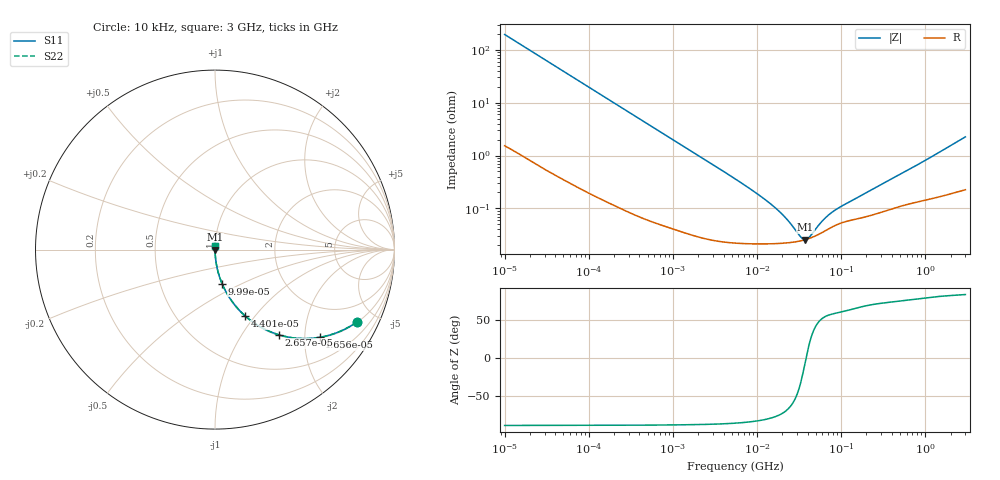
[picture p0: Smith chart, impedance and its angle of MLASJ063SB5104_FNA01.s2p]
! MLASJ063SB5104_FNA01  S-PARAMETER MODEL  ( Standard Model )
! Model Generated by TAIYO YUDEN Corporation (http://www.ty-top.com)
! Version 1.0
! TAIYO YUDEN Control No. 220601
! Copyright(c) 2005 TAIYO YUDEN CO.,LTD. All Rights Reserved.
! Product Description (link to TY-COMPAS)
! https://ds.yuden.co.jp/TYCOMPAS/or/detail?pn=MLASJ063SB5104KFNA01&u=M
! Products Name : Multilayer Ceramic Capacitors
! Characteristics :
!  Capacitance : 0.1 [uF] , Rated Voltage : 6.3 [V] , TCC : X5R
!  Case Size : 0.6 x 0.3 / 0.024 x 0.012 [mm/inch] , Thickness : 0.3 / 0.012 [mm/inch]
!  (Conditions: Temperature = 25 [degC] , DC Bias Voltage = 0 [V])
! External Node Assignments :
!  1  o---| |---o  2
! GND o---------o GND
! Frequency Range : 10kHz  -  3GHz  [ 401 STEP ]
# MHZ S RI R 50
! Freq[MHz].  S11 Real  S11 Imag  S21 Real  S21 Imag  S12 Real  S12 Imag  S22 Real  S22 Imag
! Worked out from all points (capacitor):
!   401 points, 10 kHz to 3 GHz, reference 50 ohm
!   read as one part in series: C = 81.3 nF near 10.65 kHz
!   lowest |Z| = 25.7 mohm at 37.48 MHz (marker M1)
!   series resonance near 38.35 MHz, so ESL is about 210 pH
!   S11 on the Smith chart (normalised r, x): 10 kHz: 1.03, -3.91; 16.56 kHz: 1.02, -2.37; 26.57 kHz: 1.01, -1.48; 44.01 kHz: 1.01, -0.90; 99.9 kHz: 1.00, -0.40; 3 GHz: 1.00, +0.04
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0.01  0.7908 -0.4028  0.2092 0.4028  0.2092 0.4028  0.7908 -0.4028
0.012083  0.7226 -0.4438  0.2774 0.4438  0.2774 0.4438  0.7226 -0.4438
0.016561  0.5831 -0.489  0.4169 0.489  0.4169 0.489  0.5831 -0.489
0.026575  0.3549 -0.4743  0.6451 0.4743  0.6451 0.4743  0.3549 -0.4743
0.044011  0.1692 -0.3706  0.8308 0.3706  0.8308 0.3706  0.1692 -0.3706
0.058452  0.1045 -0.3015  0.8955 0.3015  0.8955 0.3015  0.1045 -0.3015
0.082683  0.056 -0.2252  0.944 0.2252  0.944 0.2252  0.056 -0.2252
0.099902  0.0395 -0.1899  0.9605 0.1899  0.9605 0.1899  0.0395 -0.1899
0.234035  0.00816 -0.0842  0.9918 0.0842  0.9918 0.0842  0.00816 -0.0842
0.683653  0.00136 -0.0292  0.9986 0.0292  0.9986 0.0292  0.00136 -0.0292
5.477226  0.000233 -0.00362  0.9998 0.00362  0.9998 0.00362  0.000233 -0.00362
10.29003  0.000216 -0.00183  0.9998 0.00183  0.9998 0.00183  0.000216 -0.00183
15.99985  0.000216 -0.00105  0.9998 0.00105  0.9998 0.00105  0.000216 -0.00105
22.63272  0.000222 -0.000584  0.9998 0.000584  0.9998 0.000584  0.000222 -0.000584
33.04079  0.000243 -0.000157  0.9998 0.000157  0.9998 0.000157  0.000243 -0.000157
37.4819  0.000255 -2.38e-05  0.9997 2.38e-05  0.9997 2.38e-05  0.000255 -2.38e-05
41.20027  0.000268 7.53e-05  0.9997 -7.53e-05  0.9997 -7.53e-05  0.000268 7.53e-05
45.28751  0.000283 0.000174  0.9997 -0.000174  0.9997 -0.000174  0.000283 0.000174
62.07353  0.000363 0.000497  0.9996 -0.000497  0.9996 -0.000497  0.000363 0.000497
82.4407  0.000465 0.000771  0.9995 -0.000771  0.9995 -0.000771  0.000465 0.000771
374.4521  0.000956 0.0033  0.999 -0.0033  0.999 -0.0033  0.000956 0.0033
3000  0.00275 0.0224  0.9973 -0.0224  0.9973 -0.0224  0.00275 0.0224
